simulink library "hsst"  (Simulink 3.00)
undefined symbols (not defined in the file or in its folder): Final, l, m3, s, to
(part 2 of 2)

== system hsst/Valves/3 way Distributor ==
  Curr : Inport  Port=1  PortWidth=-1  SampleTime=-1  DataType=auto
  In_Pressures : Inport  Port=2  PortWidth=-1  SampleTime=-1  DataType=auto
  Out_Pressure : Inport  Port=3  PortWidth=-1  SampleTime=-1  DataType=auto
  In_Flows : Outport  Port=1  InitialOutput=0
  Out_Flow : Outport  Port=2  InitialOutput=0
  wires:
  ? -> Out_Flow/1
  Curr/1 -> ?
  ? -> In_Flows/1

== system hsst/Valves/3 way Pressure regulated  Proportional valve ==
  note: Servovalve Model
  Curr : Inport  Port=1  PortWidth=-1  SampleTime=-1  DataType=auto
  In_Pressures : Inport  Port=2  PortWidth=-1  SampleTime=-1  DataType=auto
  Out_Pressure : Inport  Port=3  PortWidth=-1  SampleTime=-1  DataType=auto
  In_Flow : Outport  Port=1  InitialOutput=0
  Out_Flow : Outport  Port=2  InitialOutput=0
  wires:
  Out_Pressure/1 -> ?
  ? -> Out_Flow/1
  Curr/1 -> ?
  ? -> In_Flow/1

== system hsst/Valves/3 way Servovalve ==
  note: Servovalve Model
  Curr : Inport  Port=1  PortWidth=-1  SampleTime=-1  DataType=auto
  In_Pressures : Inport  Port=2  PortWidth=-1  SampleTime=-1  DataType=auto
  Out_Pressure : Inport  Port=3  PortWidth=-1  SampleTime=-1  DataType=auto
  In_Flows : Outport  Port=1  InitialOutput=0
  Out_Flow : Outport  Port=2  InitialOutput=0
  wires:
  ? -> In_Flows/1
  Curr/1 -> ?
  ? -> Out_Flow/1

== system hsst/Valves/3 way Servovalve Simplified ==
  note: Servovalve Model
  Curr : Inport  Port=1  PortWidth=-1  SampleTime=-1  DataType=auto
  In_Pressures : Inport  Port=2  PortWidth=-1  SampleTime=-1  DataType=auto
  Out_Pressure : Inport  Port=3  PortWidth=-1  SampleTime=-1  DataType=auto
  In_Flows : Outport  Port=1  InitialOutput=0
  Out_Flow : Outport  Port=2  InitialOutput=0
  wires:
  ? -> In_Flows/1
  ? -> ?
  Curr/1 -> ?
  Out_Pressure/1 -> ?
  ? -> Out_Flow/1
  In_Pressures/1 -> ?

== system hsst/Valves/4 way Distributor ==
  note: Servovalve Model
  Curr : Inport  Port=1  PortWidth=-1  SampleTime=-1  DataType=auto
  In_Pressures : Inport  Port=2  PortWidth=-1  SampleTime=-1  DataType=auto
  Out_Pressures : Inport  Port=3  PortWidth=-1  SampleTime=-1  DataType=auto
  In_Flows : Outport  Port=1  InitialOutput=0
  Out_Flows : Outport  Port=2  InitialOutput=0
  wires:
  ? -> In_Flows/1
  Curr/1 -> ?
  ? -> Out_Flows/1

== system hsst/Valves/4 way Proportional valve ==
  note: Proportional valve Model
  Curr : Inport  Port=1  PortWidth=-1  SampleTime=-1  DataType=auto
  In_Pressures : Inport  Port=2  PortWidth=-1  SampleTime=-1  DataType=auto
  Out_Pressures : Inport  Port=3  PortWidth=-1  SampleTime=-1  DataType=auto
  In_Flows : Outport  Port=1  InitialOutput=0
  Out_Flows : Outport  Port=2  InitialOutput=0
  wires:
  ? -> In_Flows/1
  Curr/1 -> ?
  ? -> Out_Flows/1

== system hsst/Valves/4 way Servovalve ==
  Curr : Inport  Port=1  PortWidth=-1  SampleTime=-1  DataType=auto
  In_Pressures : Inport  Port=2  PortWidth=-1  SampleTime=-1  DataType=auto
  Out_Pressures : Inport  Port=3  PortWidth=-1  SampleTime=-1  DataType=auto
  In_Flows : Outport  Port=1  InitialOutput=0
  Out_Flows : Outport  Port=2  InitialOutput=0
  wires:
  ? -> Out_Flows/1
  Curr/1 -> ?
  ? -> In_Flows/1

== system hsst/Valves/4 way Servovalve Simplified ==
  Current : Inport  Port=1  PortWidth=-1  SampleTime=-1  DataType=auto
  In_Pressures : Inport  Port=2  PortWidth=-1  SampleTime=-1  DataType=auto
  Out_Pressures : Inport  Port=3  PortWidth=-1  SampleTime=-1  DataType=auto
  In_flows : Outport  Port=1
  Out_flows : Outport  Port=2
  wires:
  Out_Pressures/1 -> ?
  ? -> In_flows/1
  In_Pressures/1 -> ?
  ? -> Out_flows/1
  Current/1 -> ?
  ? -> ?

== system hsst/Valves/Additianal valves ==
  note: In these valves, the discharge coefficient variation with Reynolds number has been taken into account. These blocks shall be used only for simulations at low temperature conditions, to avoid execution time increasing, if not necessary. The discharge coefficient in the input data shall refer to high Reynolds numbers.
  3 way  Proportional valve with variable cd : Subsystem
  3 way Pressure regulated  Proportional valve with variable cd : Subsystem
  3 way Servovalve with variable cd : Subsystem
  4 way Proportional valve with variable cd : Subsystem
  4 way Servovalve with variable cd : Subsystem

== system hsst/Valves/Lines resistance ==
  In_Pressures : Inport  Port=1  PortWidth=-1  SampleTime=-1  DataType=auto
  Out_Pressures : Inport  Port=2  PortWidth=-1  SampleTime=-1  DataType=auto
  In_Flows : Outport  Port=1  InitialOutput=0
  Out_flows : Outport  Port=2  InitialOutput=0
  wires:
  [Q2r] -> ?
  [Q1s] -> ?
  Out_Pressures/1 -> ?
  In_Pressures/1 -> ?

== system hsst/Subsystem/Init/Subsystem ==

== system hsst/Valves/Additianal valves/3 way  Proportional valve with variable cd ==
  Curr : Inport  Port=1  PortWidth=-1  SampleTime=-1  DataType=auto
  In_Pressures : Inport  Port=2  PortWidth=-1  SampleTime=-1  DataType=auto
  Out_Pressure : Inport  Port=3  PortWidth=-1  SampleTime=-1  DataType=auto
  In_Flows : Outport  Port=1  InitialOutput=0
  Out_Flow : Outport  Port=2  InitialOutput=0
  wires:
  ? -> Out_Flow/1
  Curr/1 -> ?
  ? -> In_Flows/1

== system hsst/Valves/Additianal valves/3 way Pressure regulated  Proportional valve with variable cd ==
  Curr : Inport  Port=1  PortWidth=-1  SampleTime=-1  DataType=auto
  In_Pressures : Inport  Port=2  PortWidth=-1  SampleTime=-1  DataType=auto
  Out_Pressure : Inport  Port=3  PortWidth=-1  SampleTime=-1  DataType=auto
  In_Flow : Outport  Port=1  InitialOutput=0
  Out_Flow : Outport  Port=2  InitialOutput=0
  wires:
  ? -> Out_Flow/1
  Curr/1 -> ?
  ? -> In_Flow/1
  Out_Pressure/1 -> ?

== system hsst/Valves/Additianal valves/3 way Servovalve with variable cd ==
  Curr : Inport  Port=1  PortWidth=-1  SampleTime=-1  DataType=auto
  In_Pressures : Inport  Port=2  PortWidth=-1  SampleTime=-1  DataType=auto
  Out_Pressure : Inport  Port=3  PortWidth=-1  SampleTime=-1  DataType=auto
  In_Flows : Outport  Port=1  InitialOutput=0
  Out_Flow : Outport  Port=2  InitialOutput=0
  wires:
  ? -> In_Flows/1
  Curr/1 -> ?
  ? -> Out_Flow/1

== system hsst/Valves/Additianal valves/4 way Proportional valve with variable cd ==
  Curr : Inport  Port=1  PortWidth=-1  SampleTime=-1  DataType=auto
  In_Pressures : Inport  Port=2  PortWidth=-1  SampleTime=-1  DataType=auto
  Out_Pressures : Inport  Port=3  PortWidth=-1  SampleTime=-1  DataType=auto
  In_Flows : Outport  Port=1  InitialOutput=0
  Out_Flows : Outport  Port=2  InitialOutput=0
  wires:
  ? -> In_Flows/1
  Curr/1 -> ?
  ? -> Out_Flows/1

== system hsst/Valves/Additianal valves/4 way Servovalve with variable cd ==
  Curr : Inport  Port=1  PortWidth=-1  SampleTime=-1  DataType=auto
  In_Pressures : Inport  Port=2  PortWidth=-1  SampleTime=-1  DataType=auto
  Out_Pressures : Inport  Port=3  PortWidth=-1  SampleTime=-1  DataType=auto
  In_Flows : Outport  Port=1  InitialOutput=0
  Out_Flows : Outport  Port=2  InitialOutput=0
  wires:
  ? -> Out_Flows/1
  Curr/1 -> ?
  ? -> In_Flows/1
